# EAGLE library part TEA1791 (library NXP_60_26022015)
The TEA1791AT is a member of the new generation of Synchronous Rectifier (SR) controller ICs for switched mode power supplies. Its high level of integration allows the design of a cost-effective power supply with a very low number of external components. AAL Eindhoven MK
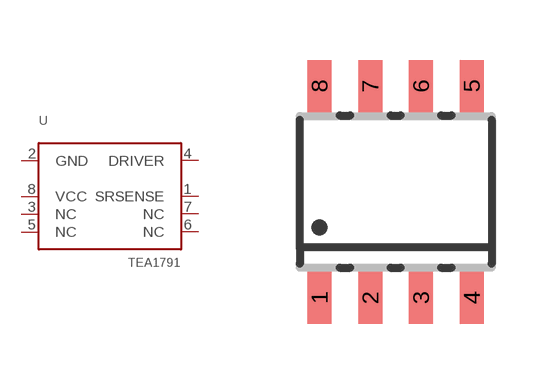
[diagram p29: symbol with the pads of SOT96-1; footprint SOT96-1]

Designator prefix U

## TEA1791AT (12NC: 9352 901 57118)  [SOT96-1]
1  SRSENSE
2  GND  pwr
3  NC
4  DRIVER  out
5  NC
6  NC
7  NC
8  VCC  pwr

## Footprint SOT96-1 (pad centres in mm)
SOT96-1 SO8: plastic small outline package; 8 leads; body width 3.9 mm JEDEC: MS-012 IEC: 076E03
smd 0.6 x 1.3: 1 -1.905,-2.65; 2 -0.635,-2.65; 3 0.635,-2.65; 4 1.905,-2.65; 5 1.905,2.65; 6 0.635,2.65; 7 -0.635,2.65; 8 -1.905,2.65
